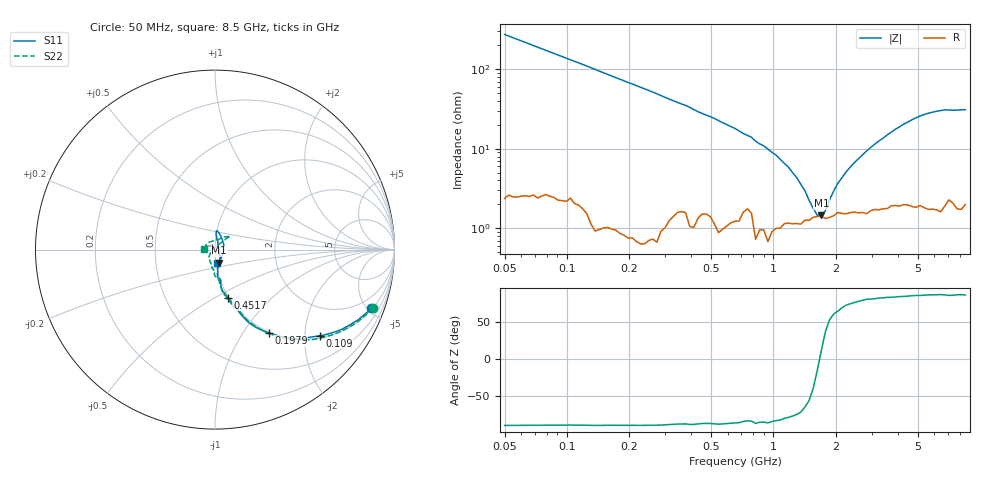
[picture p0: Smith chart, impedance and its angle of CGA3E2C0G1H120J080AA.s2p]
! S-parameter Generated by TDK Corporation
! Copyright(C) 2015 TDK Corporation.
! All Rights Reserved.
! TDK P/N: CGA3E2C0G1H120J080AA (Multilayer Ceramic Chip Capacitors)
! Property: C=12pF
! Size(LxWxT): 1.6x0.8x0.8mm, 0.063x0.031x0.031inches
! Model Type: s2p (Touchstone File Format Version 1.0)
! Frequency: DC=Yes Start=50MHz Stop=8500MHz 114points Log-sweep
! Note:
! Model Generated on Jun. 23, 2015
! Hash(MD5):
! Port Assignments:
!  1 ---| |--- 2
! Applicable Conditions:
!  Temperature = 25 degC
!  DC Bias Voltage = 0 V
!  Small Signal Operation
! Terms and conditions regarding TDK Simulation Models
! (1)This simulation model is being provided solely for informational purposes. Please refer to the specifications of the products in terms of detailed characteristics of such products.
! (2)In no event shall TDK Corporation of any of its subsidiaries be liable for any loss or damage arising, directly or indirectly,
!  From any information contained in this simulation model, including, but not limited to loss or damages arising from any inaccuracies, omissions or errors in connection with such information.
! (3)Any and all copyrights on this simulation model are owned by TDK Corporation.
!  Duplication or redistribution of this simulation model without prior written permission from TDK Corporation is prohibited.
! (4)This simulation model is subject to any modification or change without any prior notice.
! (5)Neither TDK Corporation nor any of its subsidiaries shall make any warranty, express or implied,
!  Including but not limited to the correctness, implied warranties of merchantability and fitness for a particular purpose with respect to this simulation models.
! (6)The use of this simulation model shall be deemed to have consented to the terms and conditions hereof.
# MHz S MA R 50
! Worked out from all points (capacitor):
!   113 points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, 50 MHz to 8.5 GHz, reference 50 ohm
!   read as one part in series: C = 11.6 pF near 50 MHz
!   lowest |Z| = 1.45 ohm at 1.708 GHz (marker M1)
!   series resonance near 1.674 GHz, so ESL is about 780 pH
!   S11 on the Smith chart (normalised r, x): 50 MHz: 1.11, -5.27; 109 MHz: 1.07, -2.39; 197.9 MHz: 0.98, -1.31; 451.7 MHz: 0.99, -0.57; 8.5 GHz: 1.02, -0.15
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50  0.9288 -20.6  0.3406 69.1  0.3405 69.1  0.9372 -20.2
109.0235  0.7569 -39.3  0.6086 50.4  0.609 50.4  0.7819 -38.6
119.495  0.7296 -41.8  0.6414 48.0  0.6416 48.0  0.7539 -41.3
197.8845  0.5515 -57.2  0.8063 33.5  0.8053 33.5  0.5703 -56.2
285.5811  0.4305 -66.1  0.8864 23.9  0.8853 24.1  0.4234 -65.8
451.7277  0.2766 -75.3  0.938 14.0  0.9375 14.0  0.288 -73.6
651.9202  0.2069 -80.4  0.9574 8.3  0.9555 8.3  0.1982 -82.1
1558.024  0.08582 -76.1  0.9722 -3.5  0.9725 -3.4  0.08176 -107.3
1707.669  0.07716 -72.5  0.9728 -4.6  0.9721 -4.5  0.07448 -111.8
2248.495  0.05605 -61.5  0.9708 -8.3  0.9719 -8.3  0.05326 -129.0
2701.163  0.03741 -41.8  0.972 -10.9  0.9731 -11.0  0.03699 -138.1
3099.524  0.02493 -2.6  0.9702 -13.2  0.9697 -13.2  0.0168 -163.5
3244.963  0.01969 17.7  0.9699 -14.0  0.9685 -14.1  0.00925 157.3
3397.226  0.02466 32.0  0.9705 -14.9  0.97 -14.9  0.008745 110.8
3556.634  0.03138 59.1  0.9688 -15.7  0.9683 -15.7  0.01903 69.8
3723.522  0.03715 64.5  0.9681 -16.7  0.9672 -16.7  0.02965 56.8
3898.241  0.0519 72.5  0.9663 -17.7  0.9665 -17.6  0.04071 52.0
4272.658  0.07123 82.2  0.9627 -19.6  0.9631 -19.7  0.06792 47.7
5132.831  0.1022 86.1  0.9591 -24.2  0.9569 -24.1  0.1108 41.4
6166.175  0.09386 75.4  0.956 -29.4  0.9573 -29.4  0.09885 46.8
7407.553  0.04837 -9.0  0.9531 -35.3  0.9549 -35.4  0.04928 103.6
8500  0.07373 -79.5  0.954 -41.4  0.953 -41.3  0.05866 178.0
